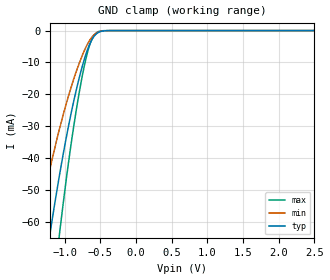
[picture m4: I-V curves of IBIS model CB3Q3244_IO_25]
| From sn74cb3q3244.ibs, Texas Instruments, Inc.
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[Model]   CB3Q3244_IO_25
Model_type  Terminator
| variable   typ   min   max
C_comp   2.82pF   2.37pF   3.05pF
| C_tri-state   2.82pF   2.37pF   3.05pF
[Temperature Range]   40   100   -40
| Ambient temperature   25   85   -40
[Voltage range]   2.5   2.3   2.7
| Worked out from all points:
|   GND clamp passes 1 mA (typ) near -0.55 V on its own axis
[GND Clamp]
| CB3Q3244_IO_25
|   Voltage   I(typ)   I(min)   I(max)
-5.5V     -958.6mA   -743.8mA   -1.181A
-1.385V   -91.56mA   -62.44mA   -128.8mA
-1.2V     -63.17mA   -42.92mA   -89.28mA
-1.08V    -46.58mA   -31.67mA   -65.55mA
-1.06V    -43.97mA   -29.92mA   -61.79mA
-920mV    -27.25mA   -18.67mA   -37.46mA
-835mV    -18.58mA   -12.8mA    -24.86mA
-755mV    -11.49mA   -7.986mA   -14.64mA
-650mV    -4.402mA   -3.123mA   -4.669mA
-550mV    -942.9uA   -723.6uA   -620.1uA
-350mV    -6.075uA   -8.963uA   -674.6nA
2.5V      246.1pA    769.2pA    127.1pA
